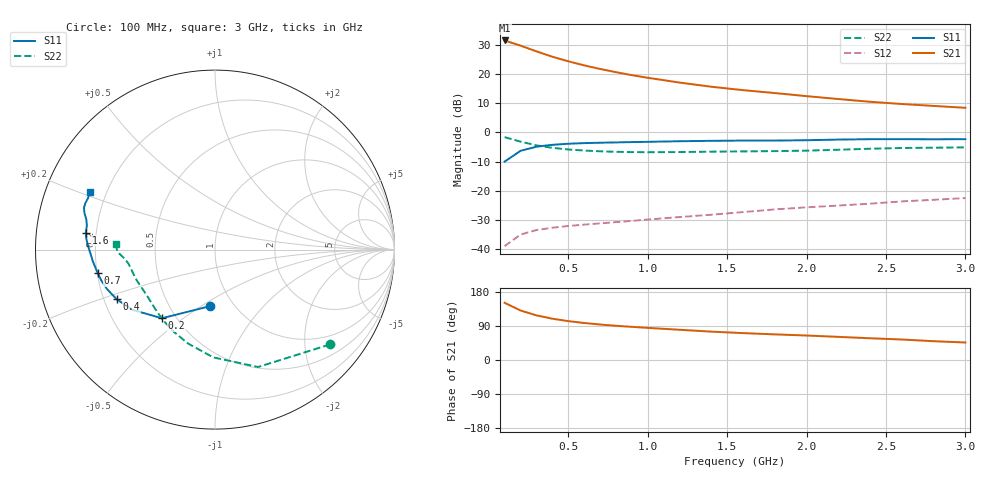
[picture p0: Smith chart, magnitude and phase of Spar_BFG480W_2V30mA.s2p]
! Filename: 230BFG480.001
! Title: BFG480W
! Bias: Vce=2V; Ic=30mA
! Company: NXP Semiconductors NL
! User: Quality&Reliability T&D
! Measure time: 10 Nov 1999 / 11:53:39
#  MHz  S  MA  R 50
! Freq  S11  S21  S12  S22  :
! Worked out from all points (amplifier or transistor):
!   20 points, 100 MHz to 3 GHz, reference 50 ohm
!   highest |S21| = 31.6 dB at 100 MHz (marker M1)
!   |S21| within 3 dB of that: start of sweep to 262.3 MHz
!   unconditionally stable (mu >= 1): 1.177 GHz to end of sweep
!   at 400 MHz: K = 0.50, MSG = 29.4 dB, |S12| = -32.8 dB
!   at 1.2 GHz: K = 1.01, MAG = 22.6 dB, |S12| = -29.1 dB
!   at 3 GHz: K = 1.14, MAG = 13.3 dB, |S12| = -22.5 dB
!   S11 on the Smith chart (normalised r, x): 100 MHz: 0.78, -0.55; 200 MHz: 0.42, -0.42; 400 MHz: 0.25, -0.22; 700 MHz: 0.20, -0.10; 1.6 GHz: 0.16, +0.06; 3 GHz: 0.14, +0.22
100  0.3158 -94.7  38.22 151.0  0.0111 67.1  0.8307 -39.5
200  0.4835 -127.7  31.14 130.7  0.01761 53.3  0.6968 -69.9
300  0.5694 -143.9  24.85 117.8  0.02097 46.9  0.6007 -90.9
400  0.6138 -153.2  20.09 109.0  0.02303 44.5  0.5445 -106.0
500  0.6404 -159.9  16.77 102.6  0.02464 44.1  0.511 -117.1
600  0.6561 -164.7  14.26 97.7  0.02603 44.4  0.4895 -125.5
700  0.6666 -168.6  12.38 93.7  0.02734 46.0  0.4752 -132.1
800  0.6749 -171.8  10.89 90.3  0.02878 47.6  0.4655 -137.6
900  0.6838 -174.6  9.685 87.5  0.03016 49.6  0.4599 -142.2
1000  0.6911 -177.2  8.728 84.8  0.03188 51.3  0.4576 -146.3
1200  0.7068 178.6  7.222 79.8  0.03515 54.4  0.4608 -153.1
1400  0.719 175.4  6.122 74.9  0.0385 56.9  0.4681 -158.2
1600  0.726 172.5  5.346 71.0  0.0428 59.4  0.473 -162.2
1800  0.7262 169.5  4.765 67.6  0.04759 61.5  0.4783 -166.1
2000  0.7361 166.8  4.217 64.6  0.05163 63.6  0.4872 -170.4
2200  0.7555 164.3  3.761 61.0  0.05541 64.6  0.5047 -174.1
2400  0.7662 162.3  3.372 57.4  0.05971 65.1  0.5258 -176.7
2600  0.7674 160.3  3.087 54.1  0.06533 65.3  0.5412 -178.4
2800  0.7633 157.9  2.862 49.6  0.0696 64.6  0.5476 179.5
3000  0.7679 155.2  2.658 46.2  0.07458 64.6  0.5542 176.6
